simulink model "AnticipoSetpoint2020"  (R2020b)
settings: Solver=ode4  StartTime=0.0  StopTime=1  FixedStep=0.0001  RelTol=1e-3  EnableMultiTasking=on
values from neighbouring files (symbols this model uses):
  tau = 0.005    [AnticipoSetpoint2020_script.m]    (also in CompDisturbiMisurabili_01_script.m = 0.01)

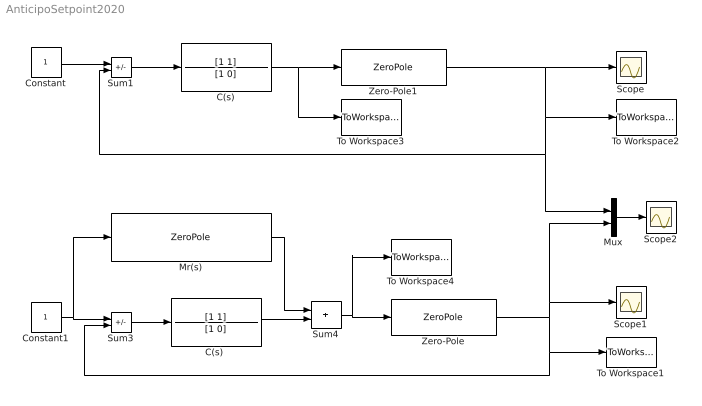
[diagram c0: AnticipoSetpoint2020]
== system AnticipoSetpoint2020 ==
  C(s) : TransferFcn  Numerator=[1 1]  Denominator=[1 0]
  "C(s) " : TransferFcn  Numerator=[1 1]  Denominator=[1 0]
  Constant : Constant
  Constant1 : Constant
  Mr(s) : ZeroPole  Zeros=[-1 -3]  Poles=[-2 -1/tau]  Gain=[1/tau]
  Mux : Mux  Inputs=2
  Scope : Scope
  Scope1 : Scope
  Scope2 : Scope
  Sum1 : Sum  Inputs=+-
  Sum3 : Sum  Inputs=+-
  Sum4 : Sum
  To Workspace1 : ToWorkspace  VariableName=yf  SaveFormat=Timeseries  SampleTime=-1
  To Workspace2 : ToWorkspace  VariableName=y  SaveFormat=Timeseries  SampleTime=-1
  To Workspace3 : ToWorkspace  VariableName=u  SaveFormat=Timeseries  SampleTime=-1
  To Workspace4 : ToWorkspace  VariableName=uf  SaveFormat=Timeseries  SampleTime=-1
  Zero-Pole : ZeroPole  Zeros=[-2]  Poles=[-1 -3]
  Zero-Pole1 : ZeroPole  Zeros=[-2]  Poles=[-1 -3]
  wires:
  C(s)/1 -> To Workspace3/1, Zero-Pole1/1
  Sum1/1 -> C(s)/1
  Zero-Pole1/1 -> Scope/1, Mux/1, Sum1/2, To Workspace2/1
  Constant/1 -> Sum1/1
  Sum3/1 -> "C(s) "/1
  Zero-Pole/1 -> Mux/2, Scope1/1, To Workspace1/1, Sum3/2
  "C(s) "/1 -> Sum4/2
  Constant1/1 -> Mr(s)/1, Sum3/1
  Mux/1 -> Scope2/1
  Sum4/1 -> To Workspace4/1, Zero-Pole/1
  Mr(s)/1 -> Sum4/1
